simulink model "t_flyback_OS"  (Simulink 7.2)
settings: Solver=ode3  SolverMode=SingleTasking  StartTime=0.0  StopTime=0.02  FixedStep=10e-6  MaxStep=5e-6  RelTol=1e-6  AbsTol=1e-6

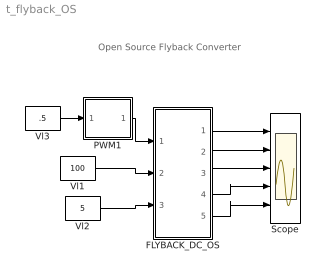
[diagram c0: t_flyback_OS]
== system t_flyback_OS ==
  note: Open Source Flyback Converter
  FLYBACK_DC_OS : Subsystem  mask{L1=1e-3, L2=4*1e-3, KP=1, C=1e-4, UC0=200, R=5}
      mask prompts: L1 "Inductance L1"; L2 "Inductance L2"; KP "Coupling Coeff"; C "Cap"; UC0 "initial Cap Voltage"; R "Load Resistance"
      mask help: Open Source Flyback Converter Input Vector u: u[0]= T1.gate u[1]= E.v u[2]= IDC.i Output Vector y: y[0]= T1.I y[1]= D1.I y[2]= Mut_L1.I y[3]= Mut_L1.V y[4]= Mut_L2.V y[5]= C1.V Parameter Vector p: p[0]= Mut_L1.L1 p[1]= Mut_L2.L2 p[2]= Mut_Coupling Coeff.k p[3]= C1.C p[4]= C1.vC0 p[5]= R1.r You can pause the simulation during running, change the Parameters you want and continue the Simulation
  PWM1 : Subsystem  mask(PWMtr){FS=1e3}
      mask prompts: FS "Frequency"
  Scope : Scope  NumInputPorts=5
  Vl1 : Constant  Value=100
  Vl2 : Constant  Value=5
  Vl3 : Constant  Value=.5
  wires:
  Vl3/1 -> PWM1/1(In1)
  PWM1/1(Out1) -> FLYBACK_DC_OS/1(sw)
  Vl1/1 -> FLYBACK_DC_OS/2(E)
  FLYBACK_DC_OS/1(iT1) -> Scope/1
  FLYBACK_DC_OS/2(iD1) -> Scope/2
  FLYBACK_DC_OS/3(tL1) -> Scope/3
  FLYBACK_DC_OS/4(vL1,vL2) -> Scope/4
  Vl2/1 -> FLYBACK_DC_OS/3(IDC)
  FLYBACK_DC_OS/5(vC) -> Scope/5

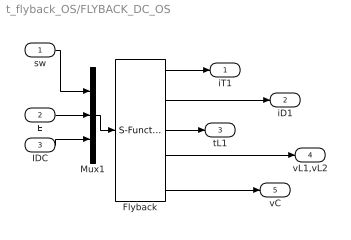
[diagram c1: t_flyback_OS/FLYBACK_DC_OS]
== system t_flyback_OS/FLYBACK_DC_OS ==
  sw : Inport  OutDataType=sfix(16)  OutScaling=2^0
  E : Inport  Port=2  OutDataType=sfix(16)  OutScaling=2^0
  IDC : Inport  Port=3  OutDataType=sfix(16)  OutScaling=2^0
  Flyback : S-Function  FunctionName=s_flyback_OS  Parameters="[L1  L2   KP  C  UC0  R]"  EnableBusSupport=off
  Mux1 : Mux  Inputs=3
  iT1 : Outport  OutDataType=sfix(16)  OutScaling=2^0
  iD1 : Outport  Port=2  OutDataType=sfix(16)  OutScaling=2^0
  tL1 : Outport  Port=3  OutDataType=sfix(16)  OutScaling=2^0
  vL1,vL2 : Outport  Port=4  OutDataType=sfix(16)  OutScaling=2^0
  vC : Outport  Port=5  OutDataType=sfix(16)  OutScaling=2^0
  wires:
  sw/1 -> Mux1/1
  E/1 -> Mux1/2
  Mux1/1 -> Flyback/1
  Flyback/1 -> iT1/1
  Flyback/2 -> iD1/1
  Flyback/3 -> tL1/1
  Flyback/4 -> vL1,vL2/1
  Flyback/5 -> vC/1
  IDC/1 -> Mux1/3

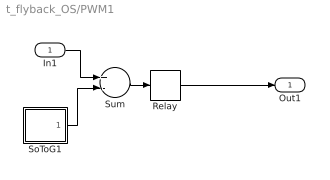
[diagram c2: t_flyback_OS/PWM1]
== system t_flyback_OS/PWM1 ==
  In1 : Inport
  Relay : Relay
  SoToG1 : Subsystem  mask(SoToG){T=1e-3}
      mask prompts: T "Period Time"
  Sum : Sum  Inputs=+-
  Out1 : Outport  InitialOutput=0
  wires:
  Relay/1 -> Out1/1
  SoToG1/1(O) -> Sum/2
  In1/1 -> Sum/1
  Sum/1 -> Relay/1

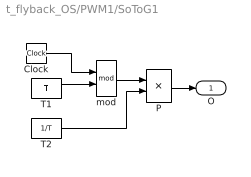
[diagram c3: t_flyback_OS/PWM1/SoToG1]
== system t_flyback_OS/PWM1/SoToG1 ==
  Clock : Clock
  P : Product
  T1 : Constant  Value=T
  T2 : Constant  Value=1/T
  mod : Math  Operator=mod
  O : Outport
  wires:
  Clock/1 -> mod/1
  T1/1 -> mod/2
  T2/1 -> P/2
  mod/1 -> P/1
  P/1 -> O/1
